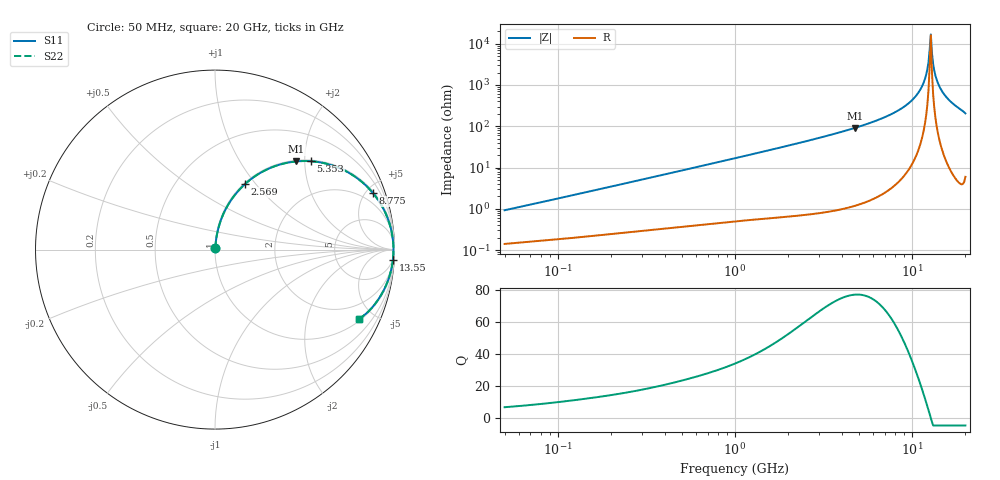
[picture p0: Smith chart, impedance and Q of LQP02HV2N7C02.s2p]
!Murata Part Number: LQP02HV2N7C02
!These Parameters are Measured in Series Mode Connection
!  o--[Z]--o
!Port1  Port2
!  o-------o
!Freq. Start=50[MHz] Stop=20[GHz], 401[Steps]
# Hz S RI R 50
!Freq.(Hz) S11(Real) S11(Imag) S21(Real) S21(Imag) S12(Real) S12(Imag) S22(Real) S22(Imag)
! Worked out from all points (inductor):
!   401 points, 50 MHz to 20 GHz, reference 50 ohm
!   read as one part in series: L = 2.87 nH near 51.52 MHz
!   highest Q = 77.2 at 4.748 GHz (marker M1), where L = 3.05 nH
!   self-resonance near 12.57 GHz
!   S11 on the Smith chart (normalised r, x): 50 MHz: 1.00, +0.02; 2.569 GHz: 1.01, +0.89; 5.353 GHz: 1.03, +2.15; 8.775 GHz: 1.11, +5.50; 13.55 GHz: 4, -34; 20 GHz: 1.12, -4.09
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5e7  0.00149 0.0091  0.9985 -0.0091  0.9985 -0.0091  0.00149 0.0091
1.364002e8  0.00264 0.0237  0.9974 -0.0237  0.9974 -0.0237  0.00264 0.0237
3.721004e8  0.00714 0.0626  0.9929 -0.0626  0.9929 -0.0626  0.00714 0.0626
1e9  0.032 0.1617  0.968 -0.1617  0.968 -0.1617  0.032 0.1617
2.569357e9  0.1681 0.3659  0.8319 -0.3659  0.8319 -0.3659  0.1681 0.3659
2.728004e9  0.1865 0.3817  0.8135 -0.3817  0.8135 -0.3817  0.1865 0.3817
4.748272e9  0.4537 0.4914  0.5463 -0.4914  0.5463 -0.4914  0.4537 0.4914
5.352748e9  0.5346 0.4923  0.4654 -0.4923  0.4654 -0.4923  0.5346 0.4923
7.442007e9  0.7727 0.4113  0.2273 -0.4113  0.2273 -0.4113  0.7727 0.4113
8.774992e9  0.8785 0.3169  0.1215 -0.3169  0.1215 -0.3169  0.8785 0.3169
1.019291e10  0.9505 0.2024  0.0495 -0.2024  0.0495 -0.2024  0.9505 0.2024
1.131968e10  0.9816 0.1102  0.0184 -0.1102  0.0184 -0.1102  0.9816 0.1102
1.201863e10  0.9911 0.0547  0.00889 -0.0547  0.00889 -0.0547  0.9911 0.0547
1.238412e10  0.9935 0.0266  0.00649 -0.0266  0.00649 -0.0266  0.9935 0.0266
1.257102e10  0.9941 0.0125  0.0059 -0.0125  0.0059 -0.0125  0.9941 0.0125
1.295331e10  0.9941 -0.0158  0.00592 0.0158  0.00592 0.0158  0.9941 -0.0158
1.314879e10  0.9935 -0.03  0.00653 0.03  0.00653 0.03  0.9935 -0.03
1.334722e10  0.9924 -0.0441  0.00755 0.0441  0.00755 0.0441  0.9924 -0.0441
1.354865e10  0.991 -0.0582  0.00898 0.0582  0.00898 0.0582  0.991 -0.0582
1.438523e10  0.9813 -0.114  0.0187 0.114  0.0187 0.114  0.9813 -0.114
1.550395e10  0.9604 -0.1815  0.0396 0.1815  0.0396 0.1815  0.9604 -0.1815
2e10  0.8002 -0.3856  0.1998 0.3856  0.1998 0.3856  0.8002 -0.3856
